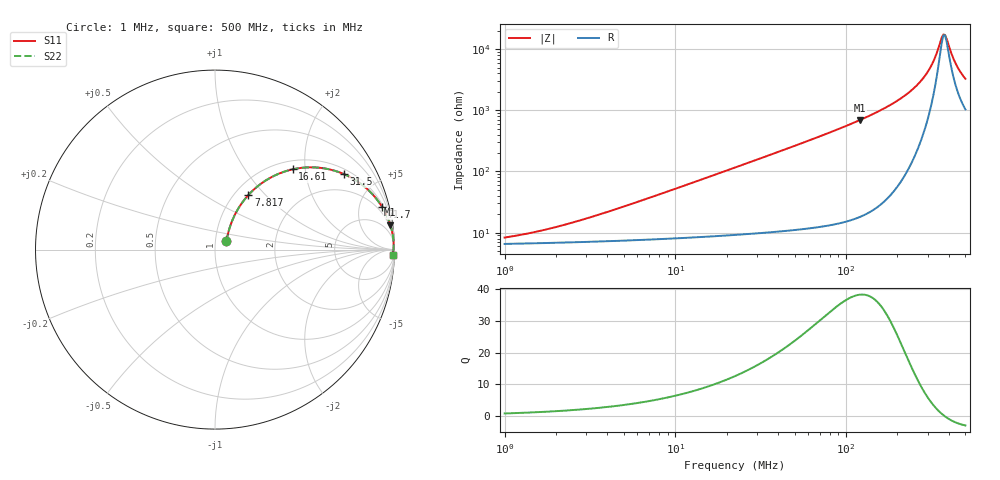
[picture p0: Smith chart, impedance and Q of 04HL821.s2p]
! Coilcraft 0402HL-821 Chip Inductor
! 20 July 2012
# MHz S MA R 50
!Freq  MagS11  AngS11  MagS21  AngS21  MagS12  AngS12  MagS22  AngS22
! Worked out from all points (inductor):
!   273 points, 1 MHz to 500 MHz, reference 50 ohm
!   read as one part in series: L = 820 nH near 4.316 MHz
!   highest Q = 38.3 at 121.3 MHz (marker M1), where L = 916 nH
!   self-resonance near 371.5 MHz
!   S11 on the Smith chart (normalised r, x): 1 MHz: 1.13, +0.10; 7.817 MHz: 1.16, +0.81; 16.61 MHz: 1.17, +1.72; 31.5 MHz: 1.20, +3.27; 71.7 MHz: 1.25, +7.67; 500 MHz: 22, -62
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1  0.07812 35.4  0.9374 -2.8  0.9374 -2.8  0.07812 35.4
1.6531  0.1015 47.0  0.9338 -4.6  0.9338 -4.6  0.1015 47.0
2.86051  0.1512 56.6  0.9255 -7.8  0.9255 -7.8  0.1512 56.6
5.064197  0.2454 60.5  0.9046 -13.7  0.9046 -13.7  0.2454 60.5
7.817026  0.3566 58.5  0.8689 -20.5  0.8689 -20.5  0.3566 58.5
7.997684  0.3635 58.3  0.8662 -20.9  0.8662 -20.9  0.3635 58.3
11.52729  0.486 53.3  0.8098 -28.8  0.8098 -28.8  0.486 53.3
16.61461  0.6226 45.9  0.7221 -38.3  0.7221 -38.3  0.6226 45.9
22.87745  0.737 38.3  0.621 -47.3  0.621 -47.3  0.737 38.3
31.50107  0.8315 30.5  0.5078 -56.1  0.5078 -56.1  0.8315 30.5
44.37777  0.9034 22.9  0.3892 -64.5  0.3892 -64.5  0.9034 22.9
63.96295  0.9503 16.2  0.2798 -71.7  0.2798 -71.7  0.9503 16.2
71.70375  0.9601 14.5  0.2502 -73.6  0.2502 -73.6  0.9601 14.5
121.2729  0.9863 8.1  0.1413 -80.4  0.1413 -80.4  0.9863 8.1
178.8336  0.9938 4.8  0.08336 -83.4  0.08336 -83.4  0.9938 4.8
235.2456  0.9958 2.9  0.04998 -83.7  0.04998 -83.7  0.9958 2.9
288.9519  0.9959 1.6  0.02761 -80.7  0.02761 -80.7  0.9959 1.6
323.9209  0.9955 0.9  0.01604 -73.1  0.01604 -73.1  0.9955 0.9
371.5139  0.9944 0.1  0.005732 -14.2  0.005732 -14.2  0.9944 0.1
380.0999  0.9942 -0.1  0.005851 8.8  0.005851 8.8  0.9942 -0.1
435.9472  0.9925 -0.8  0.01651 62.5  0.01651 62.5  0.9925 -0.8
500  0.99 -1.6  0.03023 69.9  0.03023 69.9  0.99 -1.6
